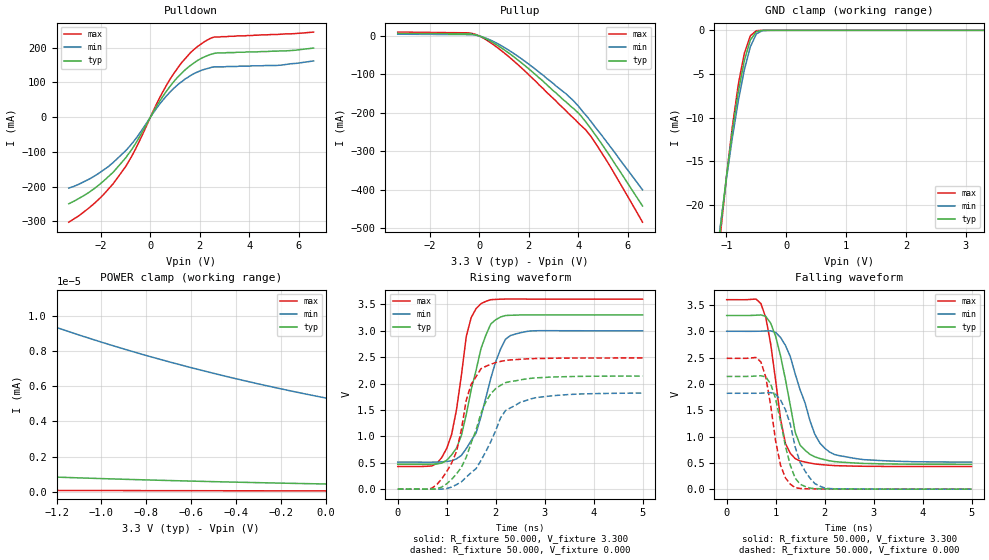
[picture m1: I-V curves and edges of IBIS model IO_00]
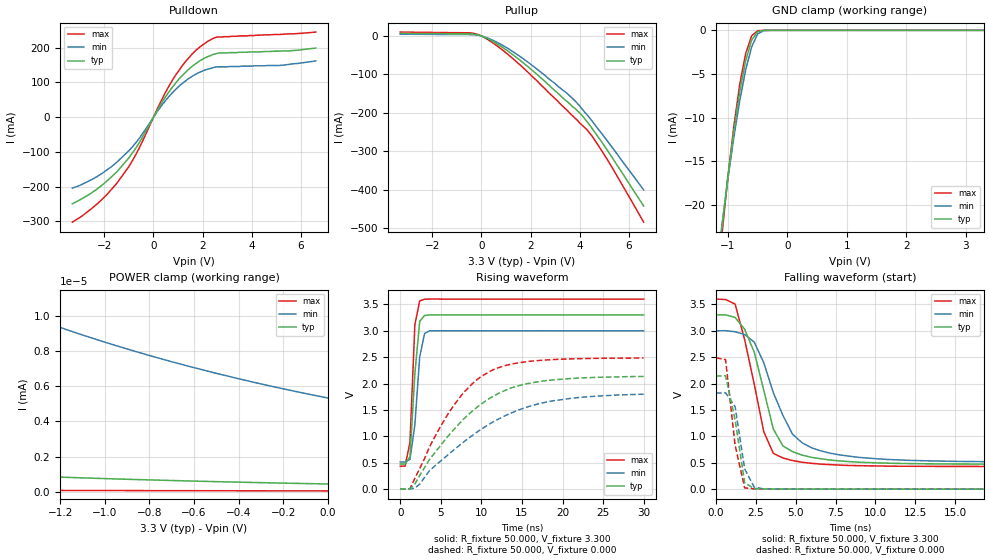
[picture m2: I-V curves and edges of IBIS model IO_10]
| / 7\'7   Xilinx XC9500 I/O Buffer IBIS File
| \ \   Xilinx Inc.
| / /   2100 Logic Drive
| \_\/.\   San Jose,   CA 95124
[IBIS ver]   3.2
[File name]   mdrive2.ibs
[File Rev]   1.3
[Date]   Fri Feb 17 00:54:48 2012
[Source]   Spice netlist
[Notes]   - max/min process data is not included in this ibis model
   - Control flag setting:
   SLW=0 - fast slew rate
   SLW=1 - slow slew rate
   VIO=0 - 3.3V Vddio
   VIO=1 - 5.0V Vddio
   NOTE: This file is compliant with IBIS Version 3.2, but it
   may not implement all approved 3.2 features.
   NOTE:  Newer versions of the buffer models may be available.
   Check the web (http://www.xilinx.com/support/sw_ibis.htm) for
   the latest file revision.  However, please be aware that the
   web files are not compatible for use with IBISWriter, and
   must be manually annotated, should their use be preferred.
[Disclaimer] The data in this model is derived from SPICE simulations
   using modeling information extracted from the target pro-
   cess. While a great deal of care has been take to provide
   information that is accurate, this model is considered
   preliminary as it has not been verified by actual silicon
   measurement. Treat the data in this model as preliminary
   until actual silicon verification is performed.
[Copyright]   Xilinx Inc.
|   Component XC9500
[Component]   XC9500
[Manufacturer]   Xilinx Inc.
[Package]
| For Package Type pc44
| variable   typ   min   max
R_pkg   0.067500m  0.066000m  0.069000m
L_pkg   3.910nH   3.550nH   4.260nH
C_pkg   0.895pF   0.790pF   1.000pF
[Pin]  signal_name   model_name   R_pin   L_pin   C_pin
5   CLK   IO_10
20   PWM   IO_10
22   CWCCW   IO_10
13   m1   IO_00
14   m2   IO_00
18   m3   IO_00
19   m4   IO_00
| Models and submodels in the file (2): IO_00 (I/O), IO_10 (I/O)
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|   Model IO_00
[Model]   IO_00
Model_type   I/O
Polarity   Non-Inverting
Enable   Active-High
Vinl =   0.800V
Vinh =   2.000V
Vmeas =   1.650V
Cref =  50.000pF
Rref =   1.000M
Vref =  0.000V
C_comp   8.000pF   6.000pF   10.000pF
[Temperature Range]   50.000   100.000   0.000
[Voltage Range]   3.300V   3.000V   3.600V
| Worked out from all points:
|   slope of the pulldown table from 0 to 0.495 V, typ, clamps not added: 8.38 ohm
|   slope of the pullup table from 0 to 0.495 V, typ, clamps not added: 32.7 ohm
|   GND clamp passes 1 mA (typ) near -0.59 V on its own axis
|   POWER clamp passes 1 mA (typ) near -2.62 V on its own axis
|   rising waveform, R_fixture 50.000, V_fixture 3.300: 20-80 % time 424ps typ, 475ps min, 314ps max; typ from 0.472 V to 3.3 V
|   rising waveform, R_fixture 50.000, V_fixture 0.000: 20-80 % time 531ps typ, 609ps min, 399ps max; typ from 0 V to 2.14 V
|   falling waveform, R_fixture 50.000, V_fixture 3.300: 20-80 % time 371ps typ, 516ps min, 300ps max; typ from 3.3 V to 0.472 V
|   falling waveform, R_fixture 50.000, V_fixture 0.000: 20-80 % time 309ps typ, 369ps min, 266ps max; typ from 2.14 V to 0 V
[Pulldown]
| voltage   I(typ)   I(min)   I(max)
-3.3V     -249mA     -204mA     -302mA
-2.3V     -207mA     -171mA     -250mA
-1.5V     -158mA     -130mA     -191mA
-1V       -117mA     -96.33mA   -142mA
-700mV    -87.07mA   -71.85mA   -105mA
300mV     37.26mA    30.59mA    45.34mA
800mV     89.38mA    72.76mA    110mA
1.3V      129mA      104mA      160mA
1.9V      163mA      130mA      203mA
2.6V      184mA      145mA      231mA
5.1V      190mA      149mA      238mA
6.6V      199mA      162mA      245mA
[Pullup]
| voltage   I(typ)   I(min)   I(max)
-3.3V     6.866mA    4.62mA     10.1mA
-300mV    4.692mA    3.207mA    6.723mA
-100mV    2.086mA    1.502mA    2.882mA
200mV     -5.344mA   -4.077mA   -7.033mA
800mV     -27.08mA   -22.04mA   -33.58mA
1.9V      -80.12mA   -68.48mA   -94.62mA
3.5V      -171mA     -150mA     -194mA
4V        -200mA     -182mA     -226mA
4.3V      -223mA     -205mA     -244mA
4.5V      -240mA     -221mA     -260mA
5.1V      -295mA     -271mA     -319mA
6.6V      -442mA     -400mA     -484mA
[GND_clamp]
| voltage   I(typ)   I(min)   I(max)
-3.3V     -211mA     -187mA     -240mA
-1.1V     -22.63mA   -22.34mA   -23.43mA
-1V       -16.78mA   -17.07mA   -16.83mA
-900mV    -11.52mA   -12.27mA   -10.99mA
-800mV    -7.005mA   -8.035mA   -6.143mA
-700mV    -3.443mA   -4.508mA   -2.631mA
-600mV    -1.112mA   -1.886mA   -628uA
-500mV    -146uA     -411uA     -39.6uA
-400mV    -11.61uA   -42.16uA   -2.469uA
-300mV    -1.054uA   -5.205uA   -140nA
3.3V      432pA      6.144nA    31.96pA
[POWER_clamp]
| voltage   I(typ)   I(min)   I(max)
-3.3V     5.154mA    7.51mA     3.331mA
-2.4V     123uA      1.138mA    24.22nA
-2.3V     13.62uA    619uA      419pA
-2.2V     550nA      241uA      105pA
-2.1V     16.36nA    51.5uA     96.67pA
-2V       1.649nA    4.929uA    92.27pA
-1.9V     1.21nA     273nA      88.15pA
-1.6V     1.022nA    11.32nA    76.95pA
-1.5V     968pA      10.78nA    73.57pA
-800mV    665pA      7.766nA    53.78pA
-400mV    536pA      6.439nA    44.83pA
0V        432pA      5.338nA    37.11pA
[Ramp]
| variable   typ   min   max
dV/dt_r   1.285/0.526n   1.092/0.632n   1.492/0.424n
dV/dt_f   1.697/0.382n   1.492/0.510n   1.902/0.286n
R_load = 50.000
[Rising Waveform]
R_fixture = 50.000
V_fixture = 3.300
V_fixture_min = 3.000
V_fixture_max = 3.600
L_fixture = 0.000H
C_fixture = 0.000F
| time   V(typ)   V(min)   V(max)
0s        472mV      512mV      430mV
700ps     474mV      511mV      440mV
1ns       546mV      524mV      772mV
1.2ns     777mV      574mV      1.503V
1.4ns     1.416V     769mV      2.892V
1.5ns     1.883V     921mV      3.251V
1.7ns     2.661V     1.374V     3.513V
2ns       3.209V     2.411V     3.595V
2.3ns     3.294V     2.909V     3.601V
5ns       3.3V       3V         3.6V
[Rising Waveform]
R_fixture = 50.000
V_fixture = 0.000
V_fixture_min = 0.000
V_fixture_max = 0.000
L_fixture = 0.000H
C_fixture = 0.000F
| time   V(typ)   V(min)   V(max)
0s        0V         0V         0V
900ps     40.2mV     570uV      196mV
1.2ns     288mV      85.05mV    711mV
1.3ns     413mV      139mV      1.126V
1.5ns     875mV      313mV      1.988V
1.7ns     1.438V     543mV      2.282V
1.9ns     1.807V     898mV      2.366V
2.2ns     2.017V     1.488V     2.437V
2.5ns     2.069V     1.645V     2.46V
5ns       2.142V     1.82V      2.486V
[Falling Waveform]
R_fixture = 50.000
V_fixture = 3.300
V_fixture_min = 3.000
V_fixture_max = 3.600
L_fixture = 0.000H
C_fixture = 0.000F
| time   V(typ)   V(min)   V(max)
0s        3.3V       3V         3.6V
700ps     3.31V      3.002V     3.525V
900ps     3.151V     3.008V     2.75V
1.1ns     2.532V     2.883V     1.332V
1.2ns     2.083V     2.732V     866mV
1.4ns     1.079V     2.187V     580mV
1.5ns     836mV      1.886V     536mV
1.8ns     614mV      1.044V     480mV
2.2ns     524mV      659mV      448mV
5ns       472mV      514mV      430mV
[Falling Waveform]
R_fixture = 50.000
V_fixture = 0.000
V_fixture_min = 0.000
V_fixture_max = 0.000
L_fixture = 0.000H
C_fixture = 0.000F
| time   V(typ)   V(min)   V(max)
0s        2.142V     1.822V     2.486V
700ps     2.155V     1.824V     2.415V
800ps     2.133V     1.829V     2.123V
900ps     1.996V     1.835V     1.583V
1.1ns     1.287V     1.693V     453mV
1.3ns     452mV      1.232V     94.06mV
1.4ns     207mV      797mV      28.25mV
1.7ns     21.29mV    211mV      6.84mV
2ns       6.649mV    23.19mV    3.202mV
5ns       11.43uV    124uV      26.53uV
|   Model IO_10
[Model]   IO_10
Model_type   I/O
Polarity   Non-Inverting
Enable   Active-High
Vinl =   0.800V
Vinh =   2.000V
Vmeas =   1.650V
Cref =  50.000pF
Rref =   1.000M
Vref =  0.000V
C_comp   8.000pF   6.000pF   10.000pF
[Temperature Range]   50.000   100.000   0.000
[Voltage Range]   3.300V   3.000V   3.600V
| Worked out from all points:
|   slope of the pulldown table from 0 to 0.495 V, typ, clamps not added: 8.38 ohm
|   slope of the pullup table from 0 to 0.495 V, typ, clamps not added: 32.7 ohm
|   GND clamp passes 1 mA (typ) near -0.59 V on its own axis
|   POWER clamp passes 1 mA (typ) near -2.62 V on its own axis
|   rising waveform, R_fixture 50.000, V_fixture 3.300: 20-80 % time 768ps typ, 784ps min, 513ps max; typ from 0.472 V to 3.3 V
|   rising waveform, R_fixture 50.000, V_fixture 0.000: 20-80 % time 7.81ns typ, 9.92ns min, 6.08ns max; typ from 0 V to 2.13 V
|   falling waveform, R_fixture 50.000, V_fixture 3.300: 20-80 % time 1.58ns typ, 2.09ns min, 1.36ns max; typ from 3.3 V to 0.472 V
|   falling waveform, R_fixture 50.000, V_fixture 0.000: 20-80 % time 733ps typ, 583ps min, 677ps max; typ from 2.14 V to 0 V
[Pulldown]
| voltage   I(typ)   I(min)   I(max)
-3.3V     -249mA     -204mA     -302mA
-2.3V     -207mA     -171mA     -250mA
-1.5V     -158mA     -130mA     -191mA
-1V       -117mA     -96.33mA   -142mA
-700mV    -87.07mA   -71.85mA   -105mA
300mV     37.26mA    30.59mA    45.34mA
800mV     89.38mA    72.75mA    110mA
1.3V      129mA      104mA      160mA
1.9V      163mA      130mA      203mA
2.6V      184mA      145mA      231mA
5.1V      190mA      149mA      238mA
6.6V      199mA      162mA      245mA
[Pullup]
| voltage   I(typ)   I(min)   I(max)
-3.3V     6.866mA    4.62mA     10.1mA
-300mV    4.692mA    3.206mA    6.723mA
-100mV    2.086mA    1.502mA    2.882mA
200mV     -5.344mA   -4.077mA   -7.033mA
800mV     -27.08mA   -22.04mA   -33.58mA
1.9V      -80.12mA   -68.48mA   -94.62mA
3.5V      -171mA     -150mA     -194mA
4V        -200mA     -182mA     -226mA
4.3V      -223mA     -205mA     -244mA
4.5V      -240mA     -221mA     -260mA
5.1V      -295mA     -271mA     -319mA
6.6V      -442mA     -400mA     -484mA
[GND_clamp]
| voltage   I(typ)   I(min)   I(max)
-3.3V     -211mA     -187mA     -240mA
-1.1V     -22.63mA   -22.34mA   -23.43mA
-1V       -16.78mA   -17.07mA   -16.83mA
-900mV    -11.52mA   -12.27mA   -10.99mA
-800mV    -7.005mA   -8.035mA   -6.143mA
-700mV    -3.443mA   -4.508mA   -2.631mA
-600mV    -1.112mA   -1.886mA   -628uA
-500mV    -146uA     -411uA     -39.6uA
-400mV    -11.61uA   -42.16uA   -2.469uA
-300mV    -1.054uA   -5.205uA   -140nA
3.3V      432pA      6.144nA    31.96pA
[POWER_clamp]
| voltage   I(typ)   I(min)   I(max)
-3.3V     5.154mA    7.51mA     3.331mA
-2.4V     123uA      1.138mA    24.22nA
-2.3V     13.62uA    619uA      419pA
-2.2V     550nA      241uA      105pA
-2.1V     16.36nA    51.5uA     96.67pA
-2V       1.649nA    4.929uA    92.27pA
-1.9V     1.21nA     273nA      88.15pA
-1.6V     1.022nA    11.32nA    76.95pA
-1.5V     968pA      10.78nA    73.57pA
-800mV    665pA      7.766nA    53.78pA
-400mV    536pA      6.439nA    44.83pA
0V        432pA      5.338nA    37.11pA
[Ramp]
| variable   typ   min   max
dV/dt_r   1.280/7.938n   1.078/9.930n   1.490/6.251n
dV/dt_f   1.697/1.613n   1.493/2.185n   1.902/1.086n
R_load = 50.000
[Rising Waveform]
R_fixture = 50.000
V_fixture = 3.300
V_fixture_min = 3.000
V_fixture_max = 3.600
L_fixture = 0.000H
C_fixture = 0.000F
| time   V(typ)   V(min)   V(max)
0s        472mV      512mV      430mV
600ps     473mV      511mV      434mV
1.2ns     608mV      561mV      888mV
1.8ns     2.181V     1.212V     3.111V
2.4ns     3.181V     2.507V     3.568V
3ns       3.29V      2.948V     3.599V
3.6ns     3.301V     3V         3.602V
30ns      3.3V       3V         3.6V
[Rising Waveform]
R_fixture = 50.000
V_fixture = 0.000
V_fixture_min = 0.000
V_fixture_max = 0.000
L_fixture = 0.000H
C_fixture = 0.000F
| time   V(typ)   V(min)   V(max)
0s        -20.61uV   -20.13uV   -10.51uV
1.2ns     80.5uV     -4.061mV   3.61mV
2.4ns     256mV      88.66mV    388mV
4.2ns     675mV      428mV      971mV
7.2ns     1.226V     815mV      1.709V
9ns       1.493V     1.027V     2.014V
11.4ns    1.752V     1.268V     2.259V
14.4ns    1.95V      1.487V     2.389V
18.6ns    2.065V     1.666V     2.452V
30ns      2.134V     1.797V     2.484V
[Falling Waveform]
R_fixture = 50.000
V_fixture = 3.300
V_fixture_min = 3.000
V_fixture_max = 3.600
L_fixture = 0.000H
C_fixture = 0.000F
| time   V(typ)   V(min)   V(max)
0s        3.3V       3V         3.6V
1.2ns     3.252V     2.981V     3.505V
1.8ns     3.029V     2.929V     2.829V
2.4ns     2.594V     2.785V     1.989V
3ns       1.868V     2.393V     1.087V
3.6ns     1.137V     1.825V     677mV
4.2ns     819mV      1.396V     591mV
5.4ns     645mV      879mV      510mV
9ns       510mV      601mV      445mV
30ns      472mV      512mV      430mV
[Falling Waveform]
R_fixture = 50.000
V_fixture = 0.000
V_fixture_min = 0.000
V_fixture_max = 0.000
L_fixture = 0.000H
C_fixture = 0.000F
| time   V(typ)   V(min)   V(max)
0s        2.142V     1.822V     2.486V
600ps     2.148V     1.824V     2.455V
1.2ns     1.313V     1.561V     833mV
1.8ns     121mV      385mV      24.09mV
2.4ns     9.881mV    36.98mV    5.526mV
3ns       4.485mV    7.228mV    3.735mV
30ns      1.589uV    4.522uV    0V
